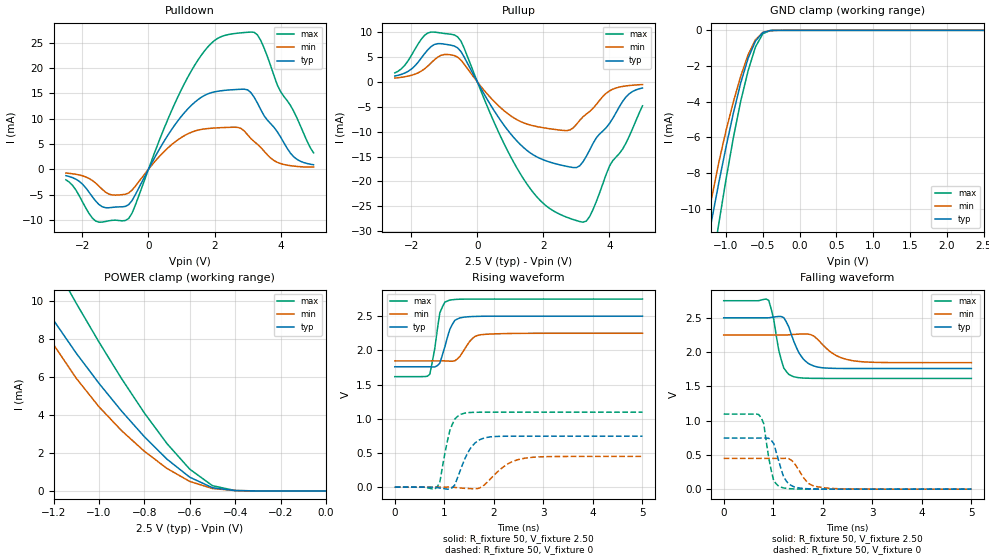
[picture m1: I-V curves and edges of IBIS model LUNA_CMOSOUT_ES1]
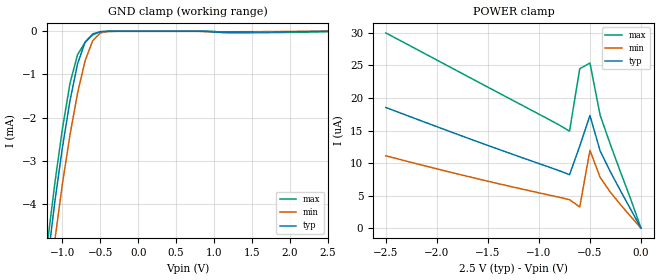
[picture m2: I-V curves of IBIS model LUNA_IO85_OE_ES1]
[IBIS Ver]   3.2
[Comment Char]   |_char
[File name]   sg-8101cx_25v_b.ibs
[File Rev]   1.0
[Date]   2018/09/14 16:40:04
[Source]
[Notes]
[Disclaimer]
This information is for modeling purposes only, and is not guaranteed.
Property of SEIKO EPSON Corp.,
unauthorized reproduction and/or distribution is strictly prohibited.
[Copyright]
Copyright 2018, SEIKO EPSON Corp.
[Component]   SG-8101CA
Si_location Pin
Timing_location Pin
[Manufacturer]   SEIKO EPSON Corp.
| 7050 PKG
| 7050 PKG
[Package]
R_pkg   224m   NA   NA
L_pkg   5.5n   NA   NA
C_pkg   0.144p   NA   NA
[Pin] signal_name   model_name
1   OE   LUNA_IO85_OE_ES1
2   VSS   GND
3   OUT   LUNA_CMOSOUT_ES1
4   VDD   POWER
[Component]   SG-8101CB
Si_location Pin
Timing_location Pin
[Manufacturer]   SEIKO EPSON Corp.
| 5032 PKG
| 5032 PKG
[Package]
R_pkg   200m   NA   NA
L_pkg   2.16n   NA   NA
C_pkg   1.23p   NA   NA
[Pin] signal_name   model_name
1   OE   LUNA_IO85_OE_ES1
2   VSS   GND
3   OUT   LUNA_CMOSOUT_ES1
4   VDD   POWER
[Component]   SG-8101CE
Si_location Pin
Timing_location Pin
[Manufacturer]   SEIKO EPSON Corp.
| 3225 PKG
| 3225 PKG
[Package]
R_pkg   177m   NA   NA
L_pkg   4.5n   NA   NA
C_pkg   0.64p   NA   NA
[Pin] signal_name   model_name
1   OE   LUNA_IO85_OE_ES1
2   VSS   GND
3   OUT   LUNA_CMOSOUT_ES1
4   VDD   POWER
[Component]   SG-8101CG
Si_location Pin
Timing_location Pin
[Manufacturer]   SEIKO EPSON Corp.
| 2520 PKG
| 2520 PKG
[Package]
R_pkg   238m   NA   NA
L_pkg   2.1n   NA   NA
C_pkg   0.38p   NA   NA
[Pin] signal_name   model_name
1   OE   LUNA_IO85_OE_ES1
2   VSS   GND
3   OUT   LUNA_CMOSOUT_ES1
4   VDD   POWER
| Models and submodels in the file (2): LUNA_CMOSOUT_ES1 (3-state), LUNA_IO85_OE_ES1 (Input)
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[Model]   LUNA_CMOSOUT_ES1
Model_type 3-state
Enable Active-High
Polarity Non-Inverting
Vmeas=1.25
C_comp   2.5p   2.0p   3.0p
[Temperature Range] 25   105   -40
[Voltage Range]   2.50   2.25   2.75
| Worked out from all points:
|   slope of the pulldown table from 0 to 0.375 V, typ, clamps not added: 84.1 ohm
|   slope of the pullup table from 0 to 0.375 V, typ, clamps not added: 85.9 ohm
|   GND clamp passes 1 mA (typ) near -0.64 V on its own axis
|   POWER clamp passes 1 mA (typ) near -0.63 V on its own axis
|   falling waveform, R_fixture 50, V_fixture 2.50: 20-80 % time 277ps typ, 421ps min, 186ps max; typ from 2.5 V to 1.76 V
|   falling waveform, R_fixture 50, V_fixture 0: 20-80 % time 199ps typ, 263ps min, 154ps max; typ from 0.745 V to 0 V
|   rising waveform, R_fixture 50, V_fixture 2.50: 20-80 % time 191ps typ, 234ps min, 144ps max; typ from 1.76 V to 2.5 V
|   rising waveform, R_fixture 50, V_fixture 0: 20-80 % time 287ps typ, 441ps min, 194ps max; typ from 0 V to 0.745 V
[Pullup]
-2.5V     1.176mA    769.1uA    1.803mA
-1.5V     6.455mA    3.18mA     9.826mA
-1.1V     7.676mA    5.339mA    9.823mA
-600mV    6.848mA    4.979mA    9.065mA
600mV     -6.731mA   -4.541mA   -9.487mA
1.5V      -13.76mA   -8.475mA   -20.51mA
2.7V      -16.97mA   -9.796mA   -27.18mA
3.2V      -16.05mA   -7.019mA   -28.2mA
3.5V      -12.4mA    -5.327mA   -25.7mA
4V        -8.373mA   -1.814mA   -16.94mA
4.5V      -3.026mA   -814.2uA   -12.31mA
5V        -1.225mA   -542uA     -4.818mA
[Pulldown]
-2.5V     -1.273mA   -752.4uA   -2.089mA
-1.6V     -6.277mA   -2.731mA   -10.23mA
-1.2V     -7.613mA   -4.908mA   -10.19mA
-600mV    -7.003mA   -4.691mA   -9.73mA
500mV     5.817mA    3.662mA    8.496mA
1.3V      12.64mA    7.311mA    19.46mA
2V        15.29mA    8.148mA    25.44mA
2.7V      15.77mA    8.275mA    26.89mA
3.3V      13.08mA    4.928mA    26.55mA
3.9V      7.422mA    1.37mA     16.68mA
4.4V      2.451mA    618.8uA    11.44mA
5V        888.7uA    420.8uA    3.235mA
[GND Clamp]
-2.5V     -55.19mA   -49.46mA   -64.23mA
-1.3V     -13.11mA   -11.85mA   -16.24mA
-1.2V     -10.77mA   -9.503mA   -13.52mA
-1.1V     -8.591mA   -7.44mA    -10.88mA
-1V       -6.541mA   -5.623mA   -8.358mA
-900mV    -4.635mA   -4.001mA   -6.009mA
-800mV    -2.939mA   -2.563mA   -3.961mA
-700mV    -1.565mA   -1.365mA   -2.263mA
-600mV    -601.2uA   -521.6uA   -925.2uA
-500mV    -121.4uA   -116.4uA   -188.8uA
-300mV    -500.8nA   -1.29uA    -313.5nA
2.5V      140pA      621.1nA    98.8pA
[POWER Clamp]
-2.5V     46.99mA    40.94mA    56.3mA
-1.4V     13.2mA     11.93mA    16.56mA
-1.3V     10.93mA    9.714mA    14.21mA
-1.2V     8.97mA     7.69mA     11.99mA
-1.1V     7.236mA    5.92mA     9.861mA
-1V       5.655mA    4.424mA    7.824mA
-900mV    4.191mA    3.162mA    5.894mA
-700mV    1.665mA    1.179mA    2.483mA
-600mV    721.7uA    498.7uA    1.143mA
-500mV    167.2uA    126.9uA    275.1uA
-400mV    16.41uA    18.75uA    19.76uA
0V        140pA      780.7pA    121.2pA
[Falling Waveform]
R_fixture=50
V_fixture=2.50
V_fixture_min=2.25
V_fixture_max=2.75
0s        2.5V       2.25V      2.75V
909.1ps   2.5V       2.25V      2.755V
1.111ns   2.52V      2.25V      2.028V
1.212ns   2.504V     2.25V      1.77V
1.414ns   2.159V     2.258V     1.64V
1.616ns   1.892V     2.265V     1.621V
1.919ns   1.779V     2.169V     1.617V
2.222ns   1.763V     1.971V     1.616V
2.626ns   1.761V     1.872V     1.616V
5ns       1.76V      1.846V     1.616V
[Falling Waveform]
R_fixture=50
V_fixture=0
V_fixture_min=0
V_fixture_max=0
0s        745.4mV    449.1mV    1.096V
707.1ps   745.4mV    449.1mV    1.09V
808.1ps   745.5mV    449.1mV    957.6mV
909.1ps   742.9mV    449.1mV    455.5mV
1.01ns    665.3mV    449.1mV    120.6mV
1.212ns   175.5mV    449.6mV    17.14mV
1.414ns   36.07mV    391.2mV    3.545mV
1.717ns   5.482mV    82.31mV    377.9uV
1.919ns   1.842mV    31.88mV    81.36uV
5ns       0V         0V         -549.9nV
[Rising Waveform]
R_fixture=50
V_fixture=2.50
V_fixture_min=2.25
V_fixture_max=2.75
0s        1.76V      1.846V     1.616V
707.1ps   1.76V      1.846V     1.651V
808.1ps   1.758V     1.846V     2.032V
909.1ps   1.812V     1.846V     2.548V
1.01ns    2.051V     1.846V     2.705V
1.111ns   2.309V     1.842V     2.735V
1.313ns   2.474V     1.91V      2.748V
1.515ns   2.493V     2.133V     2.75V
1.717ns   2.498V     2.227V     2.75V
5ns       2.5V       2.25V      2.75V
[Rising Waveform]
R_fixture=50
V_fixture=0
V_fixture_min=0
V_fixture_max=0
0s        0V         0V         0V
858.6ps   -6.799mV   -10.97uV   7.189mV
909.1ps   -13.64mV   -16.65uV   74.07mV
1.111ns   -28.61mV   736.3uV    828.7mV
1.212ns   34.33mV    -3.648mV   997.5mV
1.364ns   324.6mV    -15mV      1.072V
1.616ns   643.3mV    -23.99mV   1.094V
1.919ns   734.3mV    111mV      1.096V
2.626ns   745.4mV    423.1mV    1.096V
5ns       745.4mV    449.1mV    1.096V
[Ramp]
R_load=50
dV/dt_r   4.473E-1/2.868E-10   2.695E-1/4.402E-10   6.576E-1/1.942E-10
dV/dt_f   4.437E-1/2.729E-10   2.422E-1/4.214E-10   6.803E-1/1.778E-10
|[End   LUNA_CMOSOUT_ES1
[Model]   LUNA_IO85_OE_ES1
Model_type Input
Enable Active-Low
Polarity Non-Inverting
Vinh=1.93
Vinl=0.67
C_comp   2.5p   2.0p   3.0p
[Temperature Range] 25   105   -40
[Voltage Range]   2.50   2.25   2.75
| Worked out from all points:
|   GND clamp passes 1 mA (typ) near -0.83 V on its own axis
[GND Clamp]
-2.5V     -32.2mA    -31.31mA   -34.3mA
-1.2V     -5.408mA   -6.351mA   -4.953mA
-1.1V     -3.959mA   -4.854mA   -3.533mA
-1V       -2.702mA   -3.543mA   -2.264mA
-900mV    -1.611mA   -2.406mA   -1.207mA
-800mV    -755.7uA   -1.435mA   -544uA
-700mV    -251.7uA   -679.9uA   -254uA
-600mV    -60.42uA   -218.4uA   -84.78uA
-500mV    -8.306uA   -39.73uA   -10.67uA
-400mV    -801.3nA   -4.121uA   -821nA
1.2V      -21.43uA   -11.22uA   -36.93uA
2.5V      102pA      4.547uA    -9.898uA
[POWER Clamp]
-2.5V     18.55uA    11.12uA    30.01uA
-1.6V     13.28uA    7.586uA    22.5uA
-900mV    9.38uA     5.089uA    16.69uA
-700mV    8.214uA    4.376uA    14.9uA
-600mV    12.61uA    3.264uA    24.49uA
-500mV    17.33uA    11.98uA    25.38uA
-400mV    11.86uA    7.796uA    17.35uA
-300mV    8.666uA    5.523uA    12.86uA
-100mV    2.864uA    1.778uA    4.438uA
0V        101.8pA    233pA      102.9pA
